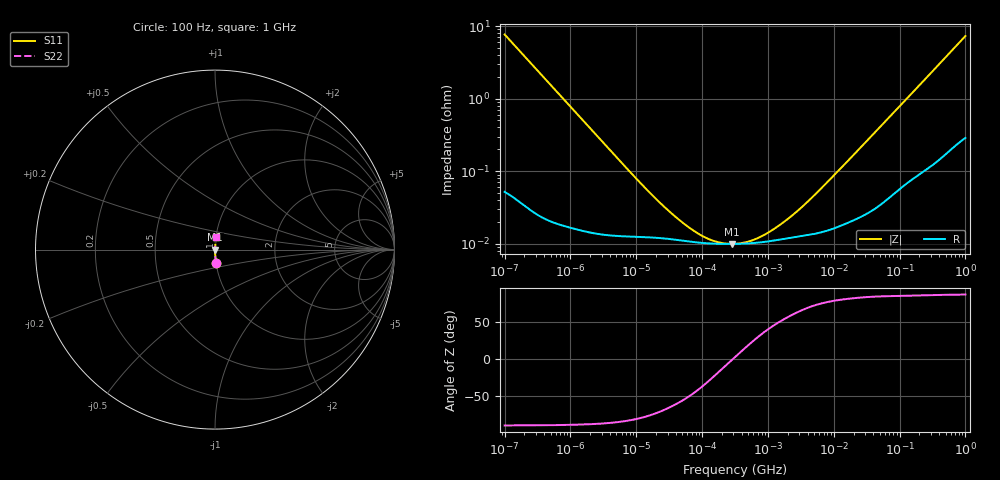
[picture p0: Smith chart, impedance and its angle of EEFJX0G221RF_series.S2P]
!  *** S-Parameter ***
!  Copyright (C) Panasonic Industry Corporation
!  Conductive Polymer Aluminum Electrolytic Capacitor (SP-Cap)
!  Parts No. EEFJX0G221RF
!  Connection Mode : Series
!  1  o---||---o  2
!  GND o--------o GND
!  Conditions : Temperature = 20   DC Bias = 0 V
! Frequency Range : 100Hz  -  1GHz  [ 401 Steps ]
# Hz S RI R 50
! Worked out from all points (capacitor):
!   401 points, 100 Hz to 1 GHz, reference 50 ohm
!   read as one part in series: C = 208 uF near 108.4 Hz
!   lowest |Z| = 9.95 mohm at 280.2 kHz (marker M1)
!   series resonance near 290.4 kHz, so ESL is about 1.4 nH
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100  0.00633 -0.076  0.9937 0.076  0.9937 0.076  0.00633 -0.076
108.3927  0.00545 -0.0702  0.9945 0.0702  0.9945 0.0702  0.00545 -0.0702
296.8247  0.000929 -0.0259  0.9991 0.0259  0.9991 0.0259  0.000929 -0.0259
1487.647  0.000178 -0.0052  0.9998 0.0052  0.9998 0.0052  0.000178 -0.0052
9120.108  0.000126 -0.000855  0.9999 0.000855  0.9999 0.000855  0.000126 -0.000855
22130.95  0.00012 -0.000359  0.9999 0.000359  0.9999 0.000359  0.00012 -0.000359
47588.28  0.000111 -0.000172  0.9999 0.000172  0.9999 0.000172  0.000111 -0.000172
94406.09  0.000103 -8.29e-05  0.9999 8.29e-05  0.9999 8.29e-05  0.000103 -8.29e-05
125169.9  0.000101 -5.75e-05  0.9999 5.75e-05  0.9999 5.75e-05  0.000101 -5.75e-05
165958.7  0.0001 -3.61e-05  0.9999 3.61e-05  0.9999 3.61e-05  0.0001 -3.61e-05
280220.6  9.95e-05 -2.18e-06  0.9999 2.18e-06  0.9999 2.18e-06  9.95e-05 -2.18e-06
316227.8  9.96e-05 5.24e-06  0.9999 -5.24e-06  0.9999 -5.24e-06  9.96e-05 5.24e-06
419276  0.0001 2.29e-05  0.9999 -2.29e-05  0.9999 -2.29e-05  0.0001 2.29e-05
555904.3  0.000102 4.21e-05  0.9999 -4.21e-05  0.9999 -4.21e-05  0.000102 4.21e-05
1017419  0.000108 9.38e-05  0.9999 -9.38e-05  0.9999 -9.38e-05  0.000108 9.38e-05
2187762  0.00012 0.0002  0.9999 -0.0002  0.9999 -0.0002  0.00012 0.0002
4704354  0.000135 0.000414  0.9999 -0.000414  0.9999 -0.000414  0.000135 0.000414
1.513561e7  0.00019 0.00127  0.9998 -0.00127  0.9998 -0.00127  0.00019 0.00127
6.99842e7  0.000462 0.00556  0.9995 -0.00556  0.9995 -0.00556  0.000462 0.00556
3.368992e8  0.0019 0.0252  0.9981 -0.0252  0.9981 -0.0252  0.0019 0.0252
9.225714e8  0.00719 0.0666  0.9928 -0.0666  0.9928 -0.0666  0.00719 0.0666
1e9  0.00808 0.072  0.9919 -0.072  0.9919 -0.072  0.00808 0.072
